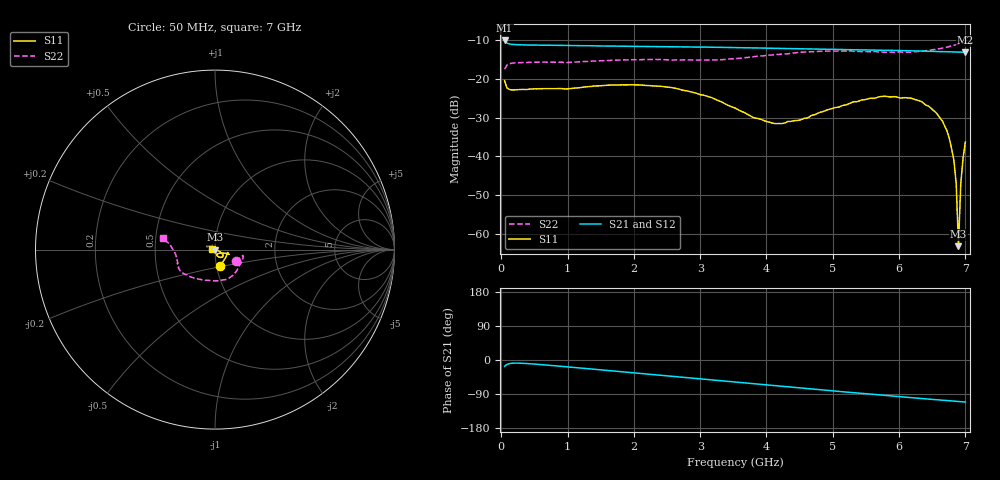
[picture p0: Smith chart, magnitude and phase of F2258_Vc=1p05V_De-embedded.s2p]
! Integrated Device Technology
! Corporate Headquarters
! 6024 Silver Creek Valley Road
! San Jose, CA 95138  USA
! Phone:  1-408-284-8200
! Toll Free:  1-800-223-1366
! Webpage:  http://www.idt.com/
! Timing and RF Division
! 515 Groton Road, Suite 102
! Westford, MA 01886-6024
! Device:  F2258
! Description: Voltage Variable RF Attenuator
! Frequency:  50.0 -  6000.00 MHz
! Package:  3x3 mm Thin QFN Plastic Package: 16 pin
! Ports:  2 RF, 2 DC
!  Pin  1  = NC
!  Pin  2  = NC
!  Pin  3  = RF2  = Port 2
!  Pin  4  = GND
!  Pin  5  = Vdd
!  Pin  6  = NC
!  Pin  7  = VCTRL
!  Pin  8  = NC
!  Pin  9  = GND
!  Pin 10  = RF1  = Port 1
!  Pin 11  = NC
!  Pin 12  = NC
!  Pin 13  = NC
!  Pin 14  = NC
!  Pin 15  = NC
!  Pin 16  = NC
! Vcntrl:  1.050 Volts
! Vdd:  +3.300 Volts
! Current:  1.159 mA
! Data:  The device was measured on a the F2258 evaluation board which has
!  individual transmission lines to the RF pins.  Data was collected
!  using a calibrated network analyzer.  The evaluation board was
!  de-embedded using a TRL calibration technique.
!  The reference plane is the edge of the package pin.
! Misc:  SN 10
!  Action Tracker AT0285
! Date Measured:  2014-12-10
! Date:  2016-01-13  MJV
! Note:
!  Integrated Device Technology supplies this data as a sample of measured
!  data at the package pin for this product.  Your particular data for this
!  product may vary.
!  Data was taken at 25 degrees C.
!  Integrated Device Technology reserves the right to change this data at anytime.
!Freq_(GHz)  S11M_(dB)  S11P_(deg)  S21M_(dB)  S21P_(deg)  S12M_(dB)  S12P_(deg)  S22M_(dB)  S22P_(deg)
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# GHz S dB R 50
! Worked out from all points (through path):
!   201 points, 50 MHz to 7 GHz, reference 50 ohm
!   highest |S21| = -10.13 dB at 50 MHz (marker M1); lowest = -13.2 dB at 7 GHz (marker M2)
!   group delay of S21, straight-line fit = 43 ps
!   lowest |S11| = -63.2 dB at 6.896 GHz (marker M3), VSWR 1.00, Z = 49.9 + j0.0237 ohm
!   |S11| at or under -10 dB: start of sweep to end of sweep
!   |S22| runs from -17.6 to -10.6 dB; largest |S21 - S12| = 0.0015
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0.05  -20.50 -72.9  -10.13 -16.6  -10.15 -16.6  -17.56 -29.9
0.08475  -22.36 -45.5  -10.80 -11.7  -10.82 -11.7  -16.50 -16.6
0.15425  -22.87 -24.8  -11.13 -8.7  -11.13 -8.7  -16.01 -12.3
1.2315  -22.20 -18.4  -11.49 -21.8  -11.47 -21.8  -15.57 -40.0
2.37825  -21.94 -17.9  -11.73 -39.8  -11.71 -39.8  -15.03 -70.2
3.07325  -24.33 -20.4  -11.84 -51.0  -11.83 -51.0  -15.18 -93.6
3.525  -27.54 -28.2  -11.97 -58.3  -11.95 -58.3  -14.82 -111.8
3.803  -30.03 -41.5  -12.06 -62.8  -12.03 -62.9  -14.31 -122.4
4.11575  -31.55 -57.4  -12.17 -67.8  -12.12 -67.8  -13.80 -132.2
4.7065  -29.33 -71.8  -12.32 -77.0  -12.30 -77.1  -13.04 -145.3
5.29725  -26.03 -59.2  -12.51 -85.9  -12.50 -86.0  -12.88 -153.7
5.85325  -24.67 -42.9  -12.68 -94.3  -12.66 -94.4  -13.18 -164.6
6.33975  -25.89 -31.5  -12.86 -101.7  -12.84 -101.7  -12.89 -176.8
6.54825  -28.61 -26.3  -12.96 -104.7  -12.95 -104.7  -12.41 177.9
6.68725  -32.16 -23.0  -13.02 -106.7  -13.01 -106.7  -11.97 174.3
6.75675  -35.31 -20.7  -13.08 -107.7  -13.06 -107.7  -11.69 172.2
6.82625  -40.99 -20.6  -13.09 -108.6  -13.08 -108.6  -11.40 171.1
6.861  -46.95 -16.7  -13.12 -109.1  -13.10 -109.1  -11.24 170.4
6.89575  -63.17 160.1  -13.14 -109.5  -13.11 -109.6  -11.04 169.6
6.9305  -46.94 168.1  -13.14 -110.0  -13.13 -110.0  -10.93 169.2
6.96525  -40.44 166.0  -13.17 -110.5  -13.14 -110.5  -10.76 168.3
7  -36.32 159.3  -13.19 -110.9  -13.15 -111.0  -10.55 167.5
